FUNCTION FC 98 : VOID
TITLE =BLOCK FOR FLY WHELL
AUTHOR : Esposito
FAMILY : TEXER
NAME : Fly_whel
VERSION : 0.1

BEGIN
NETWORK
TITLE =CONDITIONS FOR FLY WHEEL AND MISCELLANEA

NETWORK
TITLE =ALARM FLY WHEEL

NETWORK
TITLE =BIT SERVICE FLY WHEEL

NETWORK
TITLE =OPEN FLY WHEEL
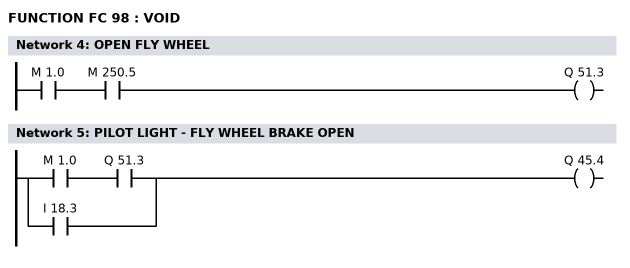
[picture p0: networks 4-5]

      A     M      1.0;
      A     M    250.5;
      =     Q     51.3;
NETWORK
TITLE =PILOT LIGHT - FLY WHEEL BRAKE OPEN

      A     M      1.0;
      A     Q     51.3;
      O     I     18.3;
      =     Q     45.4;
END_FUNCTION

